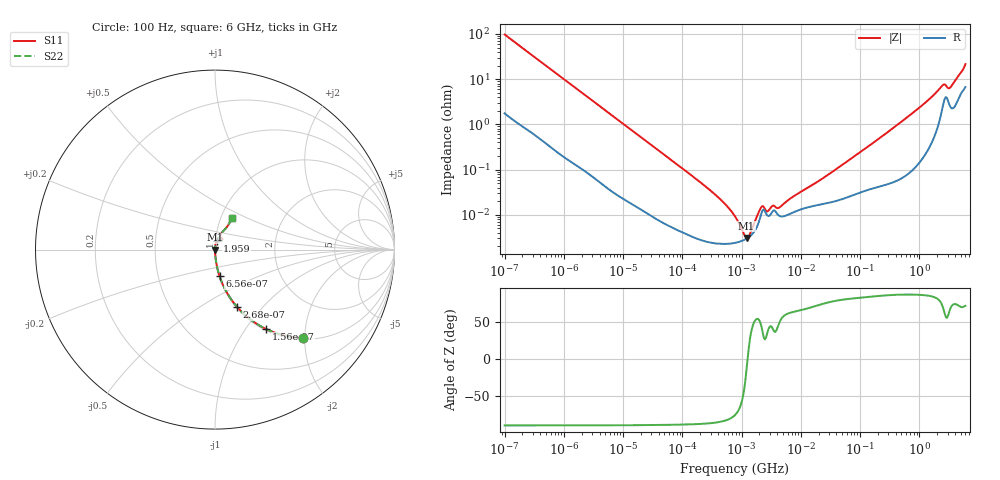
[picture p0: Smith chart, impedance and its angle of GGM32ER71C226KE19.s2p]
!Murata Part Number: GGM32ER71C226KE19
!These Parameters are Measured in Series Mode Connection
!Data Generated on Mar 13, 2026
!  o--ll--o
!Port1  Port2
!  o------o
!Operation Temp=25[degC], DC Bias Voltage=0[V]
!Freq. Start=100[Hz] Stop=6[GHz] 401[Steps]
# Hz S RI R 50
!Freq.(Hz) S11(Real) S11(Imag) S21(Real) S21(Imag) S12(Real) S12(Imag) S22(Real) S22(Imag)
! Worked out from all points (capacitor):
!   401 points, 100 Hz to 6 GHz, reference 50 ohm
!   read as one part in series: C = 16.3 uF near 109 Hz
!   lowest |Z| = 3.04 mohm at 1.212 MHz (marker M1)
!   series resonance near 1.263 MHz, so ESL is about 980 pH
!   S11 on the Smith chart (normalised r, x): 100 Hz: 1.04, -1.95; 156 Hz: 1.02, -1.25; 268 Hz: 1.01, -0.74; 656 Hz: 1.01, -0.30; 1.959 GHz: 1.01, +0.10; 6 GHz: 1.13, +0.41
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100  0.4875 -0.4909  0.5125 0.4909  0.5125 0.4909  0.4875 -0.4909
156  0.2849 -0.4425  0.7151 0.4425  0.7151 0.4425  0.2849 -0.4425
268  0.1238 -0.3201  0.8762 0.3201  0.8762 0.3201  0.1238 -0.3201
656  0.0252 -0.1477  0.9748 0.1477  0.9748 0.1477  0.0252 -0.1477
2008  0.00354 -0.05  0.9965 0.05  0.9965 0.05  0.00354 -0.05
40335  8.06e-05 -0.0026  0.9999 0.0026  0.9999 0.0026  8.06e-05 -0.0026
289253  2.44e-05 -0.000354  1 0.000354  1 0.000354  2.44e-05 -0.000354
774597  2.38e-05 -8.88e-05  1 8.88e-05  1 8.88e-05  2.38e-05 -8.88e-05
1212075  2.95e-05 -7.5e-06  1 7.5e-06  1 7.5e-06  2.95e-05 -7.5e-06
1734173  4.77e-05 6.36e-05  1 -6.36e-05  1 -6.36e-05  4.77e-05 6.36e-05
2268635  0.000126 9.15e-05  0.9999 -9.15e-05  0.9999 -9.15e-05  0.000126 9.15e-05
2713602  9.66e-05 6.8e-05  0.9999 -6.8e-05  0.9999 -6.8e-05  9.66e-05 6.8e-05
3394479  0.000122 0.000103  0.9999 -0.000103  0.9999 -0.000103  0.000122 0.000103
4246196  9.61e-05 0.000104  0.9999 -0.000104  0.9999 -0.000104  9.61e-05 0.000104
7266822  0.000111 0.000221  0.9999 -0.000221  0.9999 -0.000221  0.000111 0.000221
1.555665e7  0.000154 0.000426  0.9998 -0.000426  0.9998 -0.000426  0.000154 0.000426
3.124326e8  0.000536 0.00714  0.9995 -0.00714  0.9995 -0.00714  0.000536 0.00714
1.046602e9  0.00212 0.0244  0.9979 -0.0244  0.9979 -0.0244  0.00212 0.0244
1.95892e9  0.0098 0.0505  0.9902 -0.0505  0.9902 -0.0505  0.0098 0.0505
2.562649e9  0.0329 0.0658  0.9671 -0.0658  0.9671 -0.0658  0.0329 0.0658
3.352442e9  0.0272 0.0584  0.9728 -0.0584  0.9728 -0.0584  0.0272 0.0584
6e9  0.0961 0.1733  0.9039 -0.1733  0.9039 -0.1733  0.0961 0.1733
